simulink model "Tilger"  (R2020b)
settings: Solver=VariableStepAuto  StartTime=0.0  StopTime=100.0  RelTol=1e-3

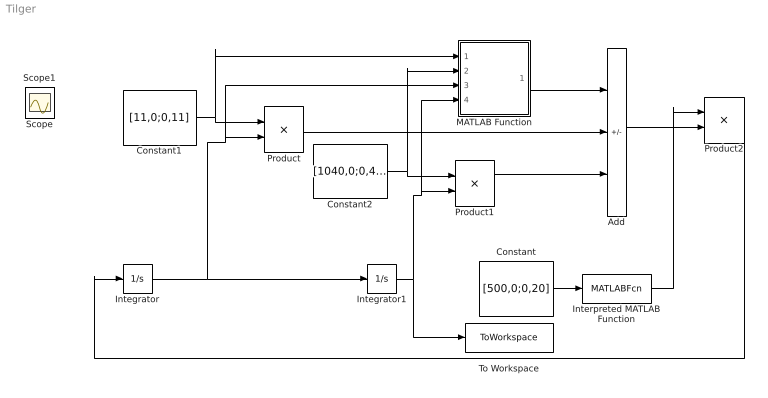
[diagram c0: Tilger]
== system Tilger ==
  Add : Sum  Inputs=+--
  Constant : Constant  Value=[500,0;0,20]  VectorParams1D=off
  Constant1 : Constant  Value=[11,0;0,11]  VectorParams1D=off
  Constant2 : Constant  Value=[1040,0;0,40]  VectorParams1D=off
  Integrator : Integrator  InitialCondition=[0;0]
  Integrator1 : Integrator  InitialCondition=[0.1;0]
  Interpreted MATLAB Function : MATLABFcn  MATLABFcn=inv(u)  Output1D=off
  MATLAB Function : MATLAB Function  TreatAsAtomicUnit=on
  Product : Product  Multiplication=Matrix(*)
  Product1 : Product  Multiplication=Matrix(*)
  Product2 : Product  Multiplication=Matrix(*)
  To Workspace : ToWorkspace  VariableName=sim  SaveFormat=Timeseries  SampleTime=-1
  Scope : Scope
  Scope1 : Scope
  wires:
  Constant1/1 -> MATLAB Function/1(D), Product/1
  Constant2/1 -> MATLAB Function/2(K), Product1/1
  Product1/1 -> Add/3
  Product/1 -> Add/2
  Constant/1 -> Interpreted MATLAB Function/1
  Interpreted MATLAB Function/1 -> Product2/1
  Product2/1 -> Integrator/1
  Add/1 -> Product2/2
  Integrator1/1 -> To Workspace/1, MATLAB Function/4(x), Product1/2
  Integrator/1 -> Integrator1/1, MATLAB Function/3(dxdt), Product/2
  MATLAB Function/1(f) -> Add/1

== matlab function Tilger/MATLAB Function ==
function f = fcn(D,K,dxdt,x)
f = [D(1,1)*dxdt(2)+K(2,2)*x(2); D(1,1)*dxdt(1)+K(2,2)*x(1)];
